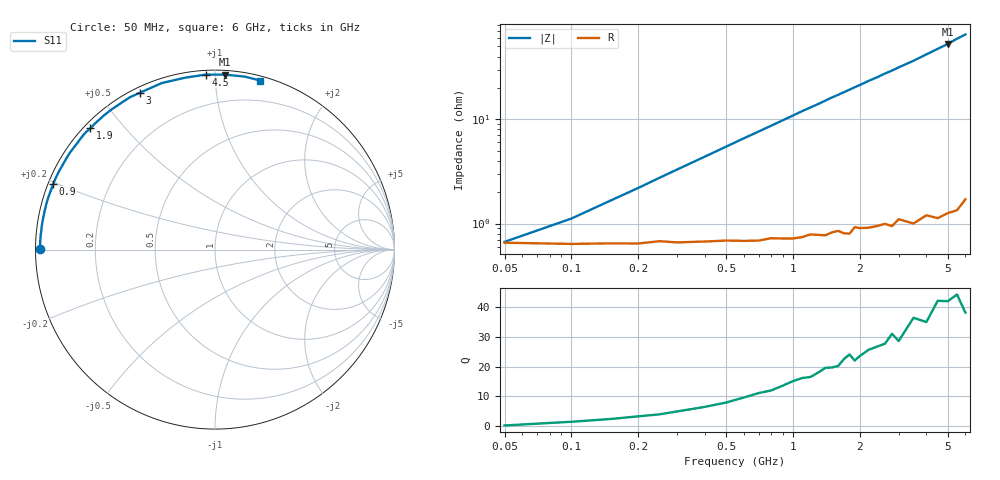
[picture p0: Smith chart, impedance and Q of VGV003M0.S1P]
! Infineon Technologies  Discrete & RF Semiconductors
! BB 831
! Si Tuning Diode in SOD323
! VR =
! S-Parameters:  July  1999
# GHz  S  MA  R  50
!  f  S11
! GHz  MAG  ANG
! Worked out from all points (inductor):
!   34 points, 50 MHz to 6 GHz, reference 50 ohm
!   read as one part to ground: L = 1.7 nH near 200 MHz
!   highest Q = 42.1 at 5 GHz (marker M1), where L = 1.68 nH
!   S11 on the Smith chart (normalised r, x): 50 MHz: 0.01, +0.00; 900 MHz: 0.01, +0.20; 1.9 GHz: 0.02, +0.41; 3 GHz: 0.02, +0.63; 4.5 GHz: 0.02, +0.95; 6 GHz: 0.03, +1.30
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0.05  0.9741 179.7
0.1  0.9748 177.9
0.15  0.9745 176.5
0.3  0.9741 172.6
0.4  0.9737 170.1
0.6  0.9735 165.1
0.7  0.9735 162.7
0.8  0.9723 160.3
0.9  0.9727 157.9
1.1  0.9723 153.1
1.3  0.9715 148.7
1.4  0.9721 146.4
1.5  0.9707 144.1
1.6  0.97 142.1
1.8  0.9725 137.9
1.9  0.9688 135.8
2  0.9698 133.9
2.2  0.9705 129.8
2.4  0.9703 126.3
2.6  0.97 122.4
2.8  0.9722 119.2
3  0.9689 115.6
3.5  0.9742 107.8
4  0.9722 100.0
4.5  0.9766 93.0
5  0.9765 86.8
5.5  0.9779 80.2
6  0.975 75.0
